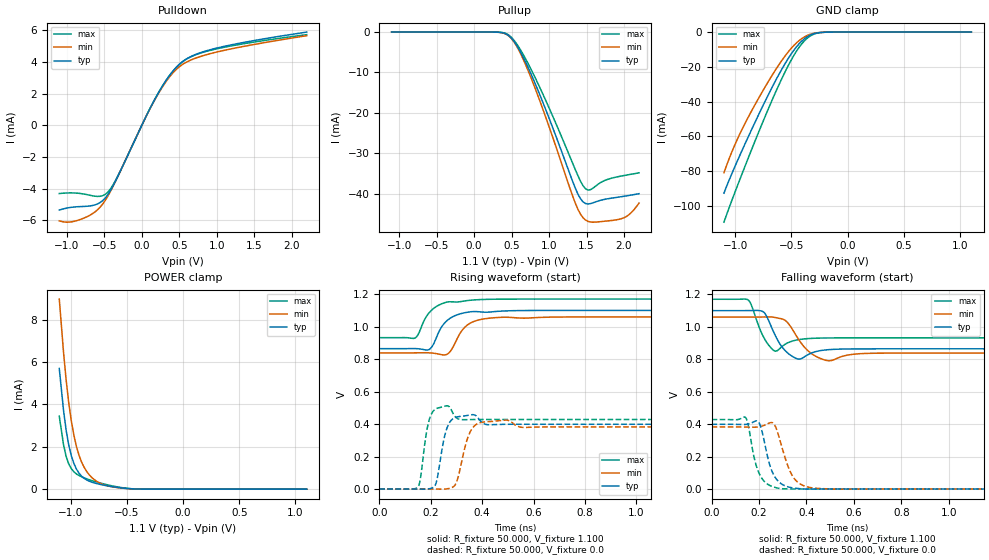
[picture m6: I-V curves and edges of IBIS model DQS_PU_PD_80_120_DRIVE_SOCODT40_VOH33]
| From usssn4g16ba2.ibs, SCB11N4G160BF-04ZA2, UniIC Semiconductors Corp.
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|   Model DQS_PU_PD_80_120_DRIVE_SOCODT40_VOH33
[Model] DQS_PU_PD_80_120_DRIVE_SOCODT40_VOH33
Model_type I/O
Polarity   Inverting
Vinl =  98.000mV
Vinh =  0.268V
Vmeas =  0.183V
Rref =  50.000
Vref =  0.183V
C_comp   1.020pF   1.010pF   1.030pF
[Model Spec]
Vinh   0.268V   0.262V   0.280V
Vinl   98.000mV   92.000mV   0.110V
Vmeas   0.183V   0.177V   0.195V
Vref   0.183V   0.177V   0.195V
Rref   50.000   NA   NA
[Temperature Range]   25.000   0.105k   -40.000
[Voltage Range]   1.100V   1.060V   1.170V
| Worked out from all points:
|   slope of the pulldown table from 0 to 0.165 V, typ, clamps not added: 105 ohm
|   GND clamp passes 1 mA (typ) near -0.30 V on its own axis
|   POWER clamp passes 1 mA (typ) near -0.95 V on its own axis
|   rising waveform, R_fixture 50.000, V_fixture 1.100: 20-80 % time 60.1ps typ, 58.2ps min, 61.2ps max; typ from 0.864 V to 1.1 V
|   rising waveform, R_fixture 50.000, V_fixture 0.0: 20-80 % time 26.1ps typ, 34.8ps min, 20.9ps max; typ from 0 V to 0.399 V
|   falling waveform, R_fixture 50.000, V_fixture 1.100: 20-80 % time 44.9ps typ, 60.8ps min, 34.8ps max; typ from 1.1 V to 0.864 V
|   falling waveform, R_fixture 50.000, V_fixture 0.0: 20-80 % time 46.3ps typ, 55.7ps min, 43.1ps max; typ from 0.399 V to 0 V
[Pulldown]
|Voltage   I(typ)   I(min)   I(max)
-1.1V     -5.34mA    -6.026mA   -4.302mA
-930mV    -5.164mA   -6.082mA   -4.26mA
-726mV    -5.101mA   -5.754mA   -4.373mA
-556mV    -4.87mA    -5.165mA   -4.475mA
-454mV    -4.386mA   -4.479mA   -4.222mA
-318mV    -3.209mA   -3.211mA   -3.18mA
192mV     1.799mA    1.766mA    1.806mA
362mV     3.096mA    3.011mA    3.096mA
532mV     3.983mA    3.811mA    3.973mA
702mV     4.448mA    4.219mA    4.427mA
1.008V    4.891mA    4.64mA     4.842mA
2.2V      5.891mA    5.665mA    5.73mA
[Pullup]
|Voltage   I(typ)   I(min)   I(max)
-1.1V     3.1nA      32.98nA    0A
432mV     -506.1uA   -571.8uA   -395uA
568mV     -3.269mA   -3.501mA   -2.92mA
704mV     -8.095mA   -8.8mA     -7.217mA
942mV     -18.54mA   -20.37mA   -16.36mA
1.316V    -37.03mA   -40.67mA   -32.54mA
1.452V    -42.01mA   -45.93mA   -38mA
1.554V    -42.45mA   -47.02mA   -39mA
1.724V    -41.47mA   -46.85mA   -36.88mA
1.962V    -40.75mA   -46.21mA   -35.64mA
2.064V    -40.44mA   -45.22mA   -35.29mA
2.2V      -40mA      -42.32mA   -34.84mA
[GND_clamp]
|Voltage   I(typ)   I(min)   I(max)
-1.1V     -92.78mA   -81.05mA   -109.5mA
-1.031V   -81.73mA   -69.22mA   -97.17mA
-939mV    -68.18mA   -56.02mA   -81.64mA
-824mV    -52mA      -41.83mA   -62.83mA
-686mV    -33.62mA   -26.41mA   -41.32mA
-571mV    -19.76mA   -15.06mA   -24.85mA
-479mV    -10.5mA    -7.76mA    -13.5mA
-410mV    -5.313mA   -3.84mA    -6.916mA
-341mV    -2.007mA   -1.45mA    -2.59mA
-272mV    -506.9uA   -403.5uA   -609.8uA
-180mV    -45.65uA   -51.35uA   -43.55uA
1.1V      0A         0A         0A
[POWER_clamp]
|Voltage   I(typ)   I(min)   I(max)
-1.1V     5.691mA    8.967mA    3.44mA
-1.062V   3.709mA    6.444mA    2.092mA
-1.039V   2.781mA    5.152mA    1.546mA
-1.016V   2.086mA    4.085mA    1.193mA
-970mV    1.21mA     2.539mA    818.5uA
-947mV    943.7uA    2.005mA    716.7uA
-901mV    610.1uA    1.27mA     581.3uA
-855mV    430.7uA    824.1uA    484.6uA
-786mV    289.9uA    439.4uA    366uA
-671mV    155.9uA    155.9uA    203.6uA
-441mV    13.2uA     12.79uA    15.03uA
1.1V      0A         0A         0A
[Ramp]
| variable   typ   min   max
dV/dt_r   0.239/26.317p   0.230/35.081p   0.257/21.178p
dV/dt_f   0.141/44.979p   0.133/60.703p   0.143/34.839p
R_load = 50.000
[Rising Waveform]
R_fixture= 50.000
V_fixture= 1.100
V_fixture_min= 1.060
V_fixture_max= 1.170
|time   V(typ)   V(min)   V(max)
0s        864.4mV    838.5mV    932.1mV
138ps     865.1mV    838.7mV    929.2mV
190ps     856.8mV    839.1mV    1.078V
205ps     876.6mV    837.5mV    1.104V
239ps     989.5mV    828.5mV    1.138V
261ps     1.034V     828mV      1.151V
280ps     1.056V     856.4mV    1.153V
329ps     1.085V     990.7mV    1.158V
385ps     1.092V     1.041V     1.166V
3ns       1.1V       1.06V      1.17V
[Rising Waveform]
R_fixture= 50.000
V_fixture= 0.0
V_fixture_min= 0.0
V_fixture_max= 0.0
|time   V(typ)   V(min)   V(max)
0s        4.355uV    15.89uV    1.03uV
152ps     -327.8uV   83.75uV    15.65mV
186ps     -258.2uV   14.4uV     370mV
212ps     11.59mV    -407.5uV   483.8mV
264ps     378.5mV    1.408mV    512.9mV
299ps     442.6mV    37.16mV    439.8mV
340ps     452.3mV    296.5mV    427.3mV
365ps     458.1mV    380.3mV    427.9mV
489ps     398.7mV    424.7mV    428.3mV
3ns       398.9mV    382.6mV    428.3mV
[Falling Waveform]
R_fixture= 50.000
V_fixture= 1.100
V_fixture_min= 1.060
V_fixture_max= 1.170
|time   V(typ)   V(min)   V(max)
0s        1.1V       1.06V      1.17V
154ps     1.1V       1.06V      1.166V
220ps     1.091V     1.061V     935mV
271ps     939.6mV    1.057V     850.2mV
315ps     846.8mV    1.034V     896.5mV
362ps     802.4mV    934.3mV    919.7mV
416ps     835.3mV    840.9mV    928.3mV
495ps     859.3mV    790.7mV    931.4mV
700ps     864.3mV    837.6mV    932.1mV
3ns       864.4mV    838.5mV    932.1mV
[Falling Waveform]
R_fixture= 50.000
V_fixture= 0.0
V_fixture_min= 0.0
V_fixture_max= 0.0
|time   V(typ)   V(min)   V(max)
0s        398.9mV    382.6mV    428.3mV
144ps     398.2mV    381.9mV    439.3mV
181ps     416.4mV    381.2mV    185.4mV
197ps     415.4mV    382.8mV    109mV
258ps     99.47mV    408mV      14.36mV
293ps     33.07mV    277.2mV    2.195mV
322ps     13.38mV    141.2mV    681.2uV
350ps     5.601mV    62.13mV    296.9uV
436ps     -434.6uV   5.052mV    23.13uV
3ns       4.147uV    15.81uV    979.4nV
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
